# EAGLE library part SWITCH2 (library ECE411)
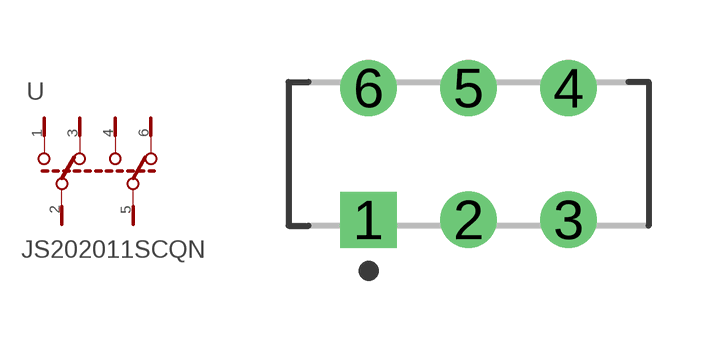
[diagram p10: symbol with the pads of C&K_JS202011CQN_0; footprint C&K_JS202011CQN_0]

Designator prefix -

## SWITCH2  [C&K_JS202011CQN_0]
1  1
2  2
3  3
4  4
5  5
6  6

## Footprint C&K_JS202011CQN_0 (pad centres in mm)
Sub-Miniature Slide Switches
drill 0.9 pad 1.4 square: 1 -2.5,-1.65
drill 0.9 pad 1.4: 2 0,-1.65; 3 2.5,-1.65; 4 2.5,1.65; 5 0,1.65; 6 -2.5,1.65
